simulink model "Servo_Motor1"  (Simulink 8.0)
settings: Solver=ode3  StartTime=0.0  StopTime=inf  RelTol=1e-3
InitFcn:
  | dt=0.01;
libraries: arduinolib x2

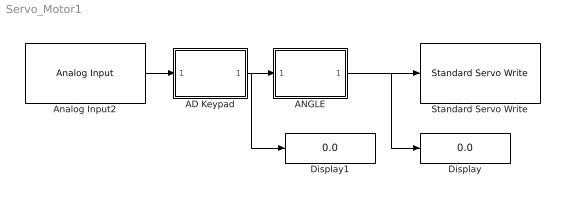
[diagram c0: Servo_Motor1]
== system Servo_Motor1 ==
  AD Keypad : MATLAB Function  TreatAsAtomicUnit=on
  ANGLE : MATLAB Function  TreatAsAtomicUnit=on
  Analog Input2 : arduinolib/Analog Input  pinNumber=1  sampleTime=dt
  Display : Display
  Display1 : Display
  Standard Servo Write : arduinolib/Standard Servo Write  pinNumber=9
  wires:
  Analog Input2/1 -> AD Keypad/1(u)
  AD Keypad/1(y) -> Display1/1, ANGLE/1(u)
  ANGLE/1(y) -> Standard Servo Write/1, Display/1

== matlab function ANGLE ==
function y = fcn(u)
persistent ang
dth=1;

if isempty(ang), ang=90; end

if u==0, ang=ang-dth; end
if u==4, ang=ang+dth; end

if ang<0, ang=0; end
if ang>180, ang=180; end

y=ang;

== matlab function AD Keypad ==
function y = fcn(u)
y=-1;
if u>=0 && u<(64-32), y=0; end
if u>=(64-32) && u<(64+32), y=1; end
if u>=(128-32) && u<(128+32), y=2; end
if u>=(192-32) && u<(192+32), y=3; end
if u>=(256-32) && u<(256+32), y=4; end
if u>=(320-32) && u<(320+32), y=5; end
if u>=(384-32) && u<(384+32), y=6; end
if u>=(448-32) && u<(448+32), y=7; end
if u>=(512-32) && u<(512+32), y=8; end
if u>=(576-32) && u<(576+32), y=9; end
if u>=(640-32) && u<(640+32), y=10; end
if u>=(704-32) && u<(704+32), y=11; end
if u>=(768-32) && u<(768+32), y=12; end
if u>=(832-32) && u<(832+32), y=13; end
if u>=(896-32) && u<(896+32), y=14; end
if u>=(960-32) && u<(960+32), y=15; end
if u<0 || u>=(960+32), y=-1; end
